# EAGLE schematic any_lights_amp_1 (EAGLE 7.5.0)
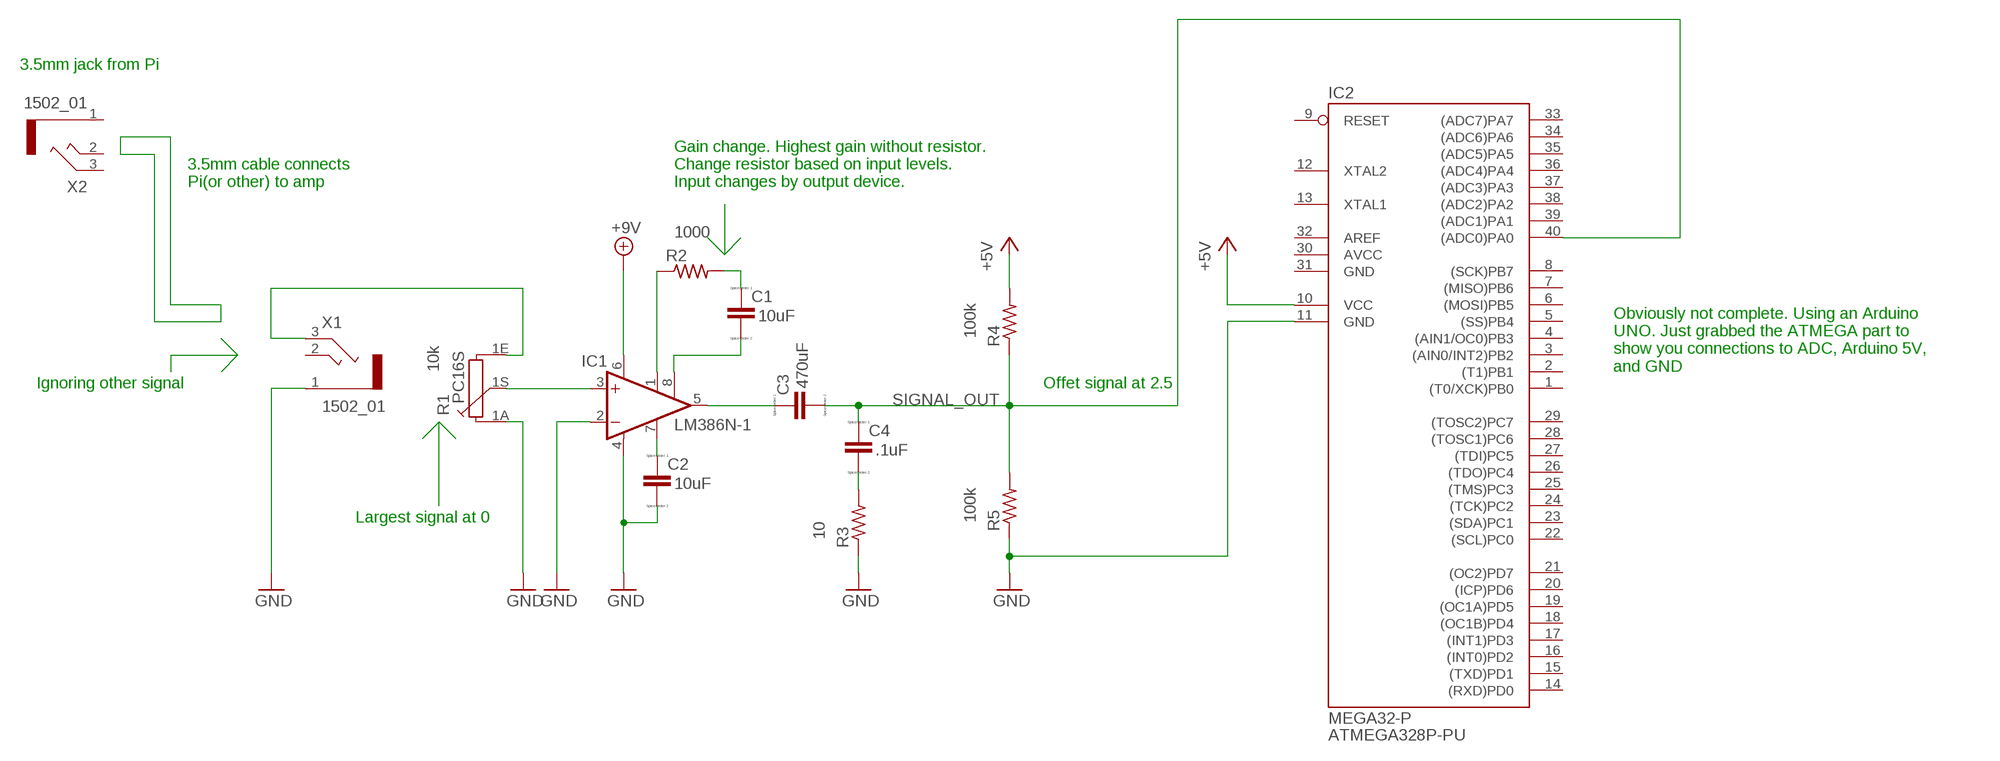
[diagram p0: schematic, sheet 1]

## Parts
C1  CC0603  [C0603]
C2  CC0603  [C0603]
C3  CC0603  [C0603]
C4  CC0603  [C0603]
IC1  LM386N-1  [DIL08]
IC2  MEGA32-P  [DIL40]
R1  PC16S  [PC16S]
R2  R-US_M0805  [M0805]
R3  R-US_M0805  [M0805]
R4  R-US_M0805  [M0805]
R5  R-US_M0805  [M0805]
X1  1502_01  [1502_01]
X2  1502_01  [1502_01]

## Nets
+5V: IC2.10(VCC) R4.2
+9V: IC1.6(VS)
GND: C2.2 IC1.2(-IN) IC1.4(GND) IC2.11(GND) R1.1A R3.1 R5.1 X1.1
N$2: R1.1E X1.3
N$3: IC1.3(+IN) R1.1S
N$4: C1.1 R2.2
N$5: IC1.1(GAIN) R2.1
N$6: C2.1 IC1.7(BYPASS)
N$7: C1.2 IC1.8(GAIN)
N$10: C3.1 IC1.5(OUT)
N$12: C4.2 R3.2
SIGNAL_OUT: C3.2 C4.1 IC2.40((ADC0)PA0) R4.1 R5.2
Unconnected: IC2.1((T0/XCK)PB0) IC2.2((T1)PB1) IC2.3((AIN0/INT2)PB2) IC2.4((AIN1/OC0)PB3) IC2.5((SS)PB4) IC2.6((MOSI)PB5) IC2.7((MISO)PB6) IC2.8((SCK)PB7) IC2.9(RESET) IC2.12(XTAL2) IC2.13(XTAL1) IC2.14((RXD)PD0) IC2.15((TXD)PD1) IC2.16((INT0)PD2) IC2.17((INT1)PD3) IC2.18((OC1B)PD4) IC2.19((OC1A)PD5) IC2.20((ICP)PD6) IC2.21((OC2)PD7) IC2.22((SCL)PC0) IC2.23((SDA)PC1) IC2.24((TCK)PC2) IC2.25((TMS)PC3) IC2.26((TDO)PC4) IC2.27((TDI)PC5) IC2.28((TOSC1)PC6) IC2.29((TOSC2)PC7) IC2.32(AREF) IC2.33((ADC7)PA7) IC2.34((ADC6)PA6) IC2.35((ADC5)PA5) IC2.36((ADC4)PA4) IC2.37((ADC3)PA3) IC2.38((ADC2)PA2) IC2.39((ADC1)PA1) X1.2 X2.1 X2.2 X2.3

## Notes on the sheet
- 3.5mm jack from Pi
- 3.5mm cable connects
  Pi(or other) to amp
- Gain change. Highest gain without resistor.
  Change resistor based on input levels.
  Input changes by output device.
- Obviously not complete. Using an Arduino
  UNO. Just grabbed the ATMEGA part to
  show you connections to ADC, Arduino 5V,
  and GND
- Ignoring other signal | Offet signal at 2.5
- Largest signal at 0

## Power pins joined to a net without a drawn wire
AVCC: IC2.30(AVCC)
GND: IC2.31(GND)

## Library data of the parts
C1 C2 = eagle-ltspice:C: CAPACITOR, European symbol; CAPACITANCE: 10uF; SPICEMODEL: NONE; SPICEPREFIX: C
C3 = eagle-ltspice:C: CAPACITOR, European symbol; CAPACITANCE: 470uF; SPICEMODEL: NONE; SPICEPREFIX: C
C4 = eagle-ltspice:C: CAPACITOR, European symbol; CAPACITANCE: .1uF; SPICEMODEL: NONE; SPICEPREFIX: C
IC1 = linear:LM386?-*: Low Voltage Audio Power Amplifier Source: http://cache.national.com/ds/LM/LM386.pdf
IC2 = atmel:MEGA32-P: MICROCONTROLLER 32 Kbytes FLASH 2 Kbytes SRAM 1 Kbytes EEPROM USART 8-channel 10 bit ADC Source: www.atmel.com .. doc2503.pdf; MPN: ATMEGA328P-PU; OC_FARNELL: 1661729; OC_NEWARK: 51P1794
R1 = piher:PC16S: POTENTIOMETER single carbon potentiometer, 16 mm, S3ROH; OC_FARNELL: 4452940; OC_NEWARK: unknown; POT_RES: 10k
R2 = resistor:R-US_: RESISTOR, American symbol; RESISTANCE: 1000
R3 = resistor:R-US_: RESISTOR, American symbol; RESISTANCE: 10
R4 R5 = resistor:R-US_: RESISTOR, American symbol; RESISTANCE: 100k
X1 X2 = con-lumberg:1502_01: Jack connectors according to JISC 6560, 3.5 mm Klinkensteckverbinder nach JISC 6560, 3,5 mm Source: http://www.lumberg.com/Produkte/PDFs/1502_01.pdf; OC_FARNELL: 4739747; OC_NEWARK: unknown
